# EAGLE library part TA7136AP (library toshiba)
PRE-AMPLIFIER FOR DUAL POWER SUPPLY VARIUOS HIGH QUALITY PRE-AMPLIFIER Source: at203a-044-ta7136ap.tif
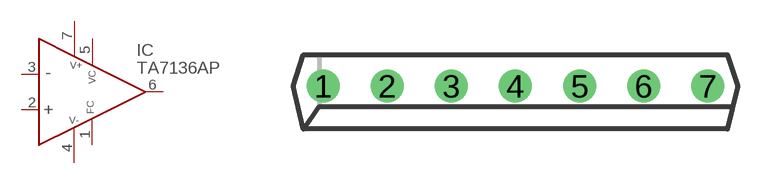
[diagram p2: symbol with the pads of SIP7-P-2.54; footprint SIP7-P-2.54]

Designator prefix IC

## TA7136AP  [SIP7-P-2.54]
1  FREQUCOMP  pas
2  +IN  in
3  -IN  in
4  V-  pwr
5  VOLTCOMP  pas
6  OUT  out
7  V+  pwr

## Footprint SIP7-P-2.54 (pad centres in mm)
SIP7-2.54 5-18A Source: THOSHIBA .. TA7136AP / at203a-044-ta7136ap.tif
drill 0.8 pad 1.27: 1 -7.62,0; 2 -5.08,0; 3 -2.54,0; 4 0,0; 5 2.54,0; 6 5.08,0; 7 7.62,0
